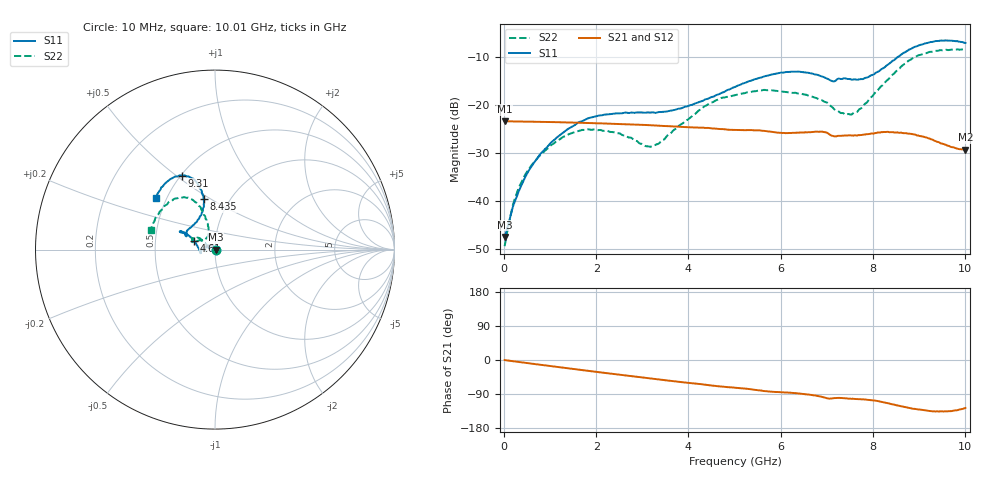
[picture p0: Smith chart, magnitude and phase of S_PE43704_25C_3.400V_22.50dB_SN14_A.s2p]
! Device ID: PE43704
! Dir: z:\PE43704\PE43704_Char_1_20130516\PE43704\AMB\3p400V\22p50dB
! Serial: 14
! Insertion: A
! Impedance: 50 ohm
! Temp: Amb
! VDD: 3.400V
! Attenuation Step: 22.50dB
! IDD: 1.140828e-01mA
#  Hz  S  RI  R  50
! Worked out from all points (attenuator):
!   401 points, 10 MHz to 10.01 GHz, reference 50 ohm
!   highest |S21| = -23.43 dB at 10 MHz (marker M1); lowest = -29.3 dB at 10.01 GHz (marker M2)
!   lowest |S11| = -47.5 dB at 10 MHz (marker M3), VSWR 1.01, Z = 50.4 + j0.0376 ohm
!   |S11| at or under -10 dB: start of sweep to 8.554 GHz
!   |S22| runs from -49.4 to -8.5 dB; largest |S21 - S12| = 0.00088
!   S11 on the Smith chart (normalised r, x): 10 MHz: 1.01, +0.00; 4.61 GHz: 0.79, +0.08; 8.435 GHz: 0.76, +0.46; 9.31 GHz: 0.51, +0.52; 10.01 GHz: 0.44, +0.31
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1e7  0.00422 0.000373  0.0674 -0.000161  0.0674 -0.000225  0.00337 0.000462
2.35e8  0.00212 0.00976  0.0669 -0.00457  0.067 -0.00454  0.00182 0.0105
5.35e8  -0.00688 0.0196  0.066 -0.01  0.066 -0.01  -0.00641 0.0205
1.085e9  -0.0366 0.0227  0.0631 -0.0196  0.0631 -0.0196  -0.0321 0.0237
1.685e9  -0.0671 0.00607  0.0581 -0.029  0.0582 -0.0289  -0.0542 0.00753
2.46e9  -0.0795 -0.0172  0.0497 -0.0391  0.0497 -0.039  -0.0501 -0.00681
3.11e9  -0.0814 -0.0178  0.0413 -0.0457  0.0413 -0.0456  -0.0367 0.00469
3.36e9  -0.0832 -0.0116  0.0377 -0.0475  0.0377 -0.0474  -0.0373 0.0137
4.285e9  -0.1042 0.0305  0.0253 -0.0519  0.0255 -0.0519  -0.0735 0.0532
4.61e9  -0.1167 0.0487  0.0204 -0.0526  0.0206 -0.0525  -0.091 0.0646
5.01e9  -0.1362 0.0699  0.0159 -0.0524  0.016 -0.0525  -0.1092 0.0625
5.585e9  -0.1679 0.0934  0.00871 -0.0532  0.00859 -0.0533  -0.1263 0.0627
5.96e9  -0.1875 0.1016  0.00467 -0.0511  0.00484 -0.0509  -0.128 0.0525
6.685e9  -0.1885 0.0954  -0.00235 -0.0522  -0.00234 -0.0519  -0.1133 0.0436
7.135e9  -0.1561 0.0793  -0.0092 -0.0466  -0.009 -0.0466  -0.0779 0.051
7.535e9  -0.1353 0.123  -0.0104 -0.0468  -0.0102 -0.0469  -0.0451 0.0647
7.86e9  -0.0959 0.1654  -0.0125 -0.0478  -0.0125 -0.0477  -0.0355 0.0978
8.36e9  -0.0618 0.2601  -0.0218 -0.047  -0.022 -0.0474  -0.0537 0.181
8.435e9  -0.0627 0.2798  -0.0236 -0.0463  -0.0236 -0.0463  -0.0631 0.1964
8.86e9  -0.1023 0.3747  -0.0307 -0.0389  -0.0302 -0.0391  -0.1235 0.2767
9.31e9  -0.1837 0.412  -0.0308 -0.0302  -0.0305 -0.0299  -0.2156 0.2855
1.001e10  -0.3285 0.2902  -0.0204 -0.0274  -0.0212 -0.0275  -0.3569 0.1109
